PROGRAM P099_Call_Recipe
VAR
	bThirdpartyHMI			: BOOL;
	iHMI: INT;
END_VAR



(*保存机器数据*)
PRG_MachineDataSave();

CASE iHMI OF

1:(*使用TwinCAT PLC HMI 操作配方*)
	PRG_Recipe_TcPlcHMI();

2:(*使用第三方触摸屏操作配方*)
	PRG_Recipe_OtherHMI();

ELSE
  (*没有配方操作的界面*)
	PRG_Recipe();

END_CASE

END_PROGRAM
